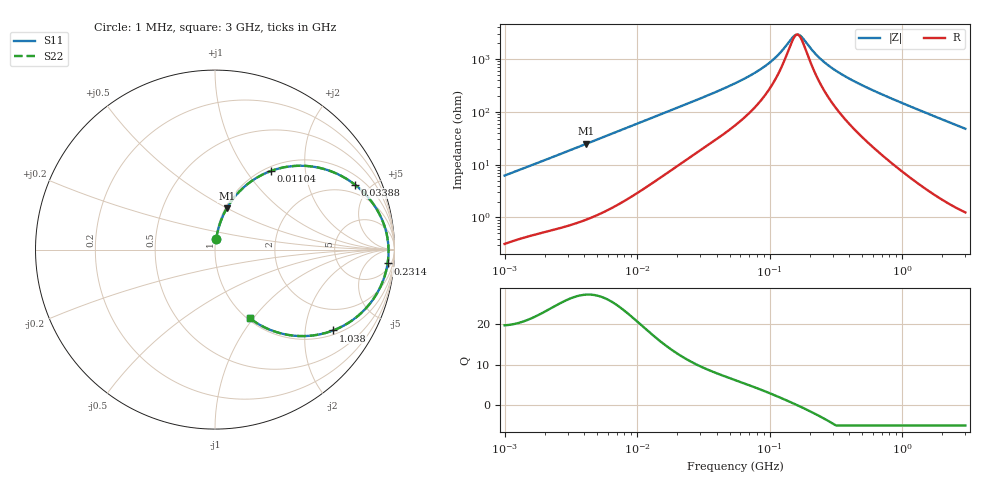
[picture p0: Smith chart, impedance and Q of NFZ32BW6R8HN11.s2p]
! NFZ32BW6R8HN11
# Hz S RI R 50
!Freq.(Hz) S11(Real) S11(Imag) S21(Real) S21(Imag) S12(Real) S12(Imag) S22(Real) S22(Imag)
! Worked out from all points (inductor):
!   401 points, 1 MHz to 3 GHz, reference 50 ohm
!   read as one part in series: L = 978 nH near 1.041 MHz
!   highest Q = 27.2 at 4.142 MHz (marker M1), where L = 954 nH
!   self-resonance near 161.4 MHz
!   S11 on the Smith chart (normalised r, x): 1 MHz: 1.01, +0.12; 11.04 MHz: 1.07, +1.32; 33.88 MHz: 1.46, +4.04; 231.4 MHz: 9, -21; 1.038 GHz: 1.14, -2.82; 3 GHz: 1.02, -0.96
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1000000  0.00695 0.0615  0.993 -0.0615  0.993 -0.0615  0.00695 0.0615
3823119  0.0571 0.2143  0.9429 -0.2143  0.9429 -0.2143  0.0571 0.2143
4141799  0.0655 0.2298  0.9345 -0.2298  0.9345 -0.2298  0.0655 0.2298
6831390  0.1526 0.3401  0.8474 -0.3401  0.8474 -0.3401  0.1526 0.3401
1.104425e7  0.3115 0.438  0.6885 -0.438  0.6885 -0.438  0.3115 0.438
1.461624e7  0.4353 0.4655  0.5647 -0.4655  0.5647 -0.4655  0.4353 0.4655
2.137957e7  0.6097 0.4484  0.3903 -0.4484  0.3903 -0.4484  0.6097 0.4484
3.387922e7  0.7802 0.3611  0.2198 -0.3611  0.2198 -0.3611  0.7802 0.3611
5.477226e7  0.8898 0.2427  0.1102 -0.2427  0.1102 -0.2427  0.8898 0.2427
7.544761e7  0.9313 0.1655  0.0687 -0.1655  0.0687 -0.1655  0.9313 0.1655
9.787053e7  0.9517 0.1065  0.0483 -0.1065  0.0483 -0.1065  0.9517 0.1065
1.171891e8  0.9603 0.0674  0.0397 -0.0674  0.0397 -0.0674  0.9603 0.0674
1.582265e8  0.9667 0.00416  0.0333 -0.00416  0.0333 -0.00416  0.9667 0.00416
1.748812e8  0.9669 -0.0169  0.0331 0.0169  0.0331 0.0169  0.9669 -0.0169
2.094008e8  0.9645 -0.0553  0.0355 0.0553  0.0355 0.0553  0.9645 -0.0553
2.314421e8  0.9617 -0.0771  0.0383 0.0771  0.0383 0.0771  0.9617 -0.0771
2.884452e8  0.9512 -0.1273  0.0488 0.1273  0.0488 0.1273  0.9512 -0.1273
3.817355e8  0.9268 -0.1964  0.0732 0.1964  0.0732 0.1964  0.9268 -0.1964
8.005644e8  0.7621 -0.3957  0.2379 0.3957  0.2379 0.3957  0.7621 -0.3957
1.038491e9  0.6582 -0.4505  0.3418 0.4505  0.3418 0.4505  0.6582 -0.4505
1.67892e9  0.4275 -0.4782  0.5725 0.4782  0.5725 0.4782  0.4275 -0.4782
3e9  0.1924 -0.3814  0.8076 0.3814  0.8076 0.3814  0.1924 -0.3814
